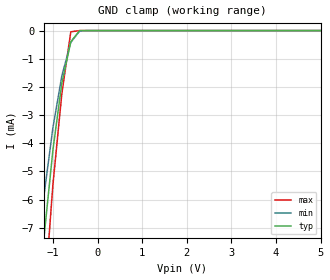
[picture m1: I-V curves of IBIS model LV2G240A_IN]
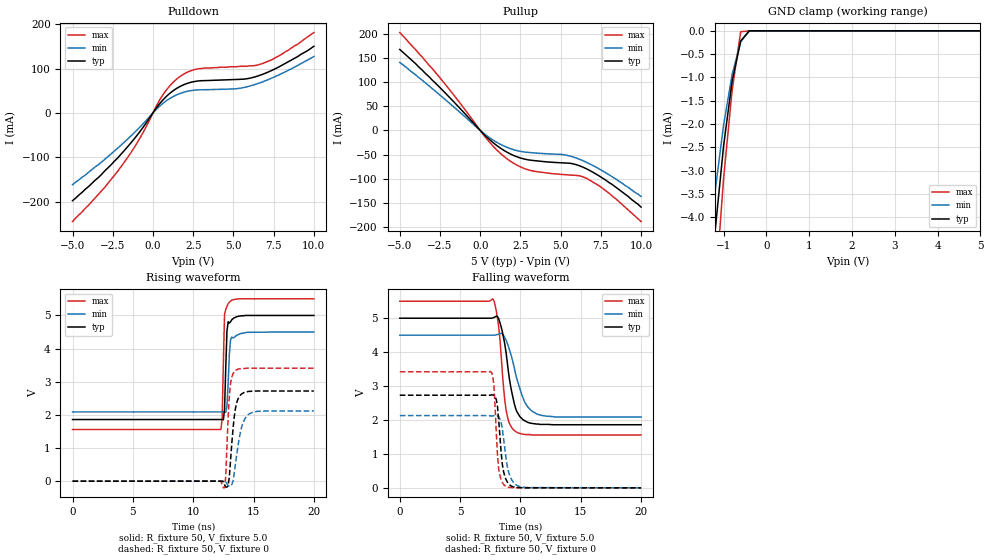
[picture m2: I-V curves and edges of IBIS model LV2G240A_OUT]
|/_/_/_/_/_/_/_/_/_/_/_/_/_/_/_/_/_/_/_/_/_/_/_/_/_/_/_/_/_/_/_/_/_/_/_/_/_/
|   Renesas Electronics Corp.
|   Multi Purpose Semiconductor Digital IC Design Group
|   IBIS Model of HD74LV2G240A
|   5.0V Dual Bus Buffer Inverted with 3-state Outputs,
|   SSOP-8(8pin) Package
|   History
|   V1.0   April   1, 2003   : First release.
|/_/_/_/_/_/_/_/_/_/_/_/_/_/_/_/_/_/_/_/_/_/_/_/_/_/_/_/_/_/_/_/_/_/_/_/_/_/
[IBIS Ver]   2.1
[Comment Char]  |_char
[File name]   l2g240s5.ibs
[File Rev]   1.1
[Date]   April 1, 2003
[Source]   Data created from SPICE simulations at
|   Renesas Electronics Corp.
[Notes]   RLC value of the Package is determined by assuming typical
|   conditions.
[Disclaimer]   This information is for modeling purposes only, and is not
|   guaranteed.
[Copyright]   Copyright 2003, Renesas Electronics Corp.,
|   All Rights Reserved.
|   Component  HD74LV2G240A
[Component]   HD74LV2G240A
[Manufacturer]  Renesas Electronics Corp.
[Package]
|   typ   min   max
R_pkg   0.099   0.095   0.102
L_pkg   1.740nH   1.680nH   1.790nH
C_pkg   0.140pF   0.140pF   0.150pF
[Pin]   signal_name   model_name   R_pin   L_pin   C_pin
1   G1   LV2G240A_IN   0.102   1.780nH   0.140pF
2   A1   LV2G240A_IN   0.097   1.710nH   0.150pF
3   Y2   LV2G240A_OUT   0.095   1.680nH   0.150pF
4   GND   GND   0.102   1.790nH   0.140pF
5   A2   LV2G240A_IN   0.101   1.790nH   0.140pF
6   Y1   LV2G240A_OUT   0.097   1.710nH   0.150pF
7   G2   LV2G240A_IN   0.097   1.710nH   0.150pF
8   VCC   POWER   0.102   1.790nH   0.140pF
| Models and submodels in the file (2): LV2G240A_IN (Input), LV2G240A_OUT (3-state)
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|   Model  LV2G240A_IN
[Model]   LV2G240A_IN
Model_type  Input
Vinl = 1.50V
Vinh = 3.50V
| variable   typ   min   max
C_comp   2.85pF   2.75pF   2.95pF
| variable   typ   min   max
[Temperature range]   25   85   -40
| variable   typ   min   max
[Voltage range]   5.0V   4.5V   5.5V
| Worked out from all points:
|   GND clamp passes 1 mA (typ) near -0.68 V on its own axis
[GND Clamp]
|   Voltage   I(typ)   I(min)   I(max)
-5V       -128mA     -106mA     -157mA
-1.4V     -11mA      -8.74mA    -14.7mA
-1.2V     -7.33mA    -5.84mA    -9.68mA
-1V       -4.23mA    -3.44mA    -5.46mA
-800mV    -1.86mA    -1.6mA     -2.23mA
-600mV    -396uA     -418uA     -43uA
-400mV    -474nA     -10.9uA    -2.94nA
5V        10.1pA     35.9pA     10pA
|   Model  LV2G240A_OUT
[Model]   LV2G240A_OUT
Model_type  3-state
Polarity   Inverting
Enable   Active-Low
Vmeas = 2.5V
| variable   typ   min   max
C_comp   8.35pF   8.25pF   8.45pF
| variable   typ   min   max
[Temperature range]   25   85   -40
| variable   typ   min   max
[Voltage range]   5.0V   4.5V   5.5V
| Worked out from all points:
|   slope of the pulldown table from 0 to 0.75 V, typ, clamps not added: 22 ohm
|   slope of the pullup table from 0 to 0.75 V, typ, clamps not added: 31.4 ohm
|   GND clamp passes 1 mA (typ) near -0.78 V on its own axis
|   rising waveform, R_fixture 50, V_fixture 5.0: 20-80 % time 160ps typ, 200ps min, 151ps max; typ from 1.86 V to 5 V
|   rising waveform, R_fixture 50, V_fixture 0: 20-80 % time 414ps typ, 601ps min, 280ps max; typ from 0 V to 2.72 V
|   falling waveform, R_fixture 50, V_fixture 5.0: 20-80 % time 858ps typ, 1.16ns min, 584ps max; typ from 5 V to 1.86 V
|   falling waveform, R_fixture 50, V_fixture 0: 20-80 % time 418ps typ, 550ps min, 321ps max; typ from 2.73 V to 0 V
[Pullup]
|   Voltage   I(typ)   I(min)   I(max)
-5V       168mA      141mA      203mA
-2.4V     85.4mA     70.5mA     105mA
200mV     -6.98mA    -5.55mA    -8.94mA
1V        -30.6mA    -24.1mA    -39.5mA
1.6V      -43.9mA    -34.1mA    -57.2mA
2.4V      -56.1mA    -42.7mA    -74mA
3.2V      -62mA      -46.2mA    -83.6mA
5.2V      -67.4mA    -50.4mA    -91.6mA
5.8V      -69.5mA    -55.3mA    -92.9mA
6.6V      -79.5mA    -66.1mA    -99.3mA
8V        -108mA     -91.8mA    -130mA
10V       -159mA     -137mA     -189mA
[Pulldown]
|   Voltage   I(typ)   I(min)   I(max)
-5V       -198mA     -162mA     -245mA
-3V       -131mA     -105mA     -168mA
-2.2V     -102mA     -79.8mA    -132mA
-800mV    -41.7mA    -31.6mA    -56.4mA
600mV     28.4mA     20.9mA     39.7mA
1V        42.6mA     31.4mA     59.1mA
1.6V      57.9mA     42.5mA     79.9mA
2.8V      71.9mA     51.8mA     99.3mA
5.2V      75.3mA     54.5mA     104mA
6.8V      86.7mA     69.8mA     111mA
8V        107mA      88.6mA     132mA
10V       150mA      127mA      181mA
[GND Clamp]
|   Voltage   I(typ)   I(min)   I(max)
-5V       -76.6mA    -64mA      -93.9mA
-1.4V     -6.55mA    -5.21mA    -8.67mA
-1.2V     -4.33mA    -3.47mA    -5.69mA
-1V       -2.48mA    -2.03mA    -3.18mA
-800mV    -1.08mA    -936uA     -1.28mA
-600mV    -219uA     -237uA     -20.5uA
-400mV    -248nA     -6.13uA    -1.4nA
5V        5.14pA     37.3pA     5pA
[Ramp]
| variable   typ   min   max
dV/dt_r   1.636/417.6p   1.276/603.6p   2.049/281.6p
dV/dt_f   1.881/855.2p   1.446/1.167n   2.363/585.4p
R_load = 50ohms
[Rising Waveform]
R_fixture = 50
V_fixture = 5.0
V_fixture_min = 4.5
V_fixture_max = 5.5
C_fixture = 0p
|   Time   V(typ)   V(min)   V(max)
0s        1.86V      2.09V      1.56V
12.3ns    1.86V      2.09V      1.56V
12.4ns    1.86V      2.09V      1.89V
12.6ns    2.17V      2.08V      5.03V
12.8ns    4.53V      2.27V      5.27V
12.9ns    4.81V      2.97V      5.36V
13ns      4.77V      3.83V      5.4V
13.1ns    4.81V      4.27V      5.43V
13.2ns    4.87V      4.35V      5.46V
20ns      5V         4.5V       5.5V
[Rising Waveform]
R_fixture = 50
V_fixture = 0
C_fixture = 0p
|   Time   V(typ)   V(min)   V(max)
0s        -203nV     258nV      579nV
12.6ns    -112mV     4.67mV     -200mV
12.7ns    -176mV     -11.3mV    149mV
13ns      135mV      -157mV     2.58V
13.1ns    641mV      -140mV     2.96V
13.4ns    1.93V      229mV      3.3V
13.6ns    2.36V      775mV      3.36V
14ns      2.63V      1.61V      3.4V
14.6ns    2.71V      2.02V      3.41V
20ns      2.72V      2.12V      3.41V
[Falling Waveform]
R_fixture = 50
V_fixture = 5.0
V_fixture_min = 4.5
V_fixture_max = 5.5
C_fixture = 0p
|   Time   V(typ)   V(min)   V(max)
0s        5V         4.5V       5.5V
7.7ns     5.01V      4.5V       5.57V
8.2ns     4.98V      4.53V      4.73V
8.6ns     4.43V      4.49V      2.95V
8.9ns     3.73V      4.27V      2.13V
9.3ns     2.79V      3.82V      1.76V
9.8ns     2.19V      3.1V       1.62V
10.6ns    1.93V      2.39V      1.57V
11.8ns    1.87V      2.13V      1.56V
20ns      1.86V      2.09V      1.56V
[Falling Waveform]
R_fixture = 50
V_fixture = 0
C_fixture = 0p
|   Time   V(typ)   V(min)   V(max)
0s        2.73V      2.13V      3.42V
7.6ns     2.74V      2.12V      3.4V
7.8ns     2.73V      2.13V      3.01V
8ns       2.6V       2.14V      1.62V
8.2ns     1.99V      2.09V      551mV
8.5ns     690mV      1.73V      159mV
8.8ns     249mV      877mV      38.5mV
9.2ns     61.3mV     291mV      9.58mV
10ns      6.42mV     30.3mV     1.06mV
20ns      -321nV     -1.81uV    -155nV
